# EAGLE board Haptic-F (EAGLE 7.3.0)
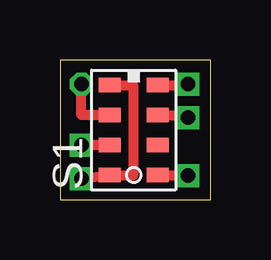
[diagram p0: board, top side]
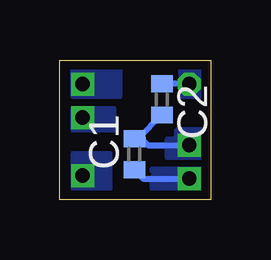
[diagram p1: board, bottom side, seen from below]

Size 6.27 x 5.83 mm. Coordinates in mm from the lower left corner, seen from the top.
Outline: 0,0 6.27,0 6.27,5.83 0,5.83 0,0
Copper layers (1*16): Top 0.0356mm / dielectric 1.5011mm / Bottom 0.0356mm
Design rules "LaenPCBOrder": minimum track width 6mil, minimum drill 13mil, track to track 6mil, track to pad 6mil, pad to pad 6mil, via to via 6mil, smd to smd 6mil, copper to edge 15mil, drill to drill 6mil, minimum pad ring 7mil, minimum via ring 7mil, stop-mask expansion 3mil, vias tented up to drill 0mil, thermal gap 10mil
Net classes: 0 default: width 0.127 mm, drill 0.508 mm, clearance 0.254 mm

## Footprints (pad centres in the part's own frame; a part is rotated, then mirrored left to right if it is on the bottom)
C0402 = smd 0.7 x 0.9: 1 -0.65,0; 2 0.65,0
LGA8 = smd 0.9 x 0.6: 1 -2.5,2.5; 2 -2.5,1.25; 3 -2.5,0; 4 -2.5,-1.25; 5 -0.5,-1.25; 6 -0.5,0; 7 -0.5,1.25; 8 -0.5,2.5

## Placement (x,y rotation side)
C1  1uf  [C0402]  3.17,1.9 90 bottom
C2  1uf  [C0402]  2.03,4.19 270 bottom
S1  MPL115A2  [LGA8]  4.57,2.29 0 top

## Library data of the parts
C1 C2 = eagle-ltspice; SPICEMODEL: NONE; SPICEPREFIX: C
S1 = Youritronics

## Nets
CAP: C2.1 S1.2
GND: C1.2 C2.2 S1.3
RST: S1.5
SCL: S1.8
SDA: S1.7
VDD: C1.1 S1.1 S1.4

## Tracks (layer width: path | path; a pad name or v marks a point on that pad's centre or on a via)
CAP  (via drill 0.6)
  Top 0.406: S1.2 0.89,3.54 v0.89,4.83
  Bottom 0.254: 0.9,4.84 C2.1
  Bottom 0.406: v0.89,4.83 0.9,4.84
  pour Bottom: 0.38,5.33 0.38,4.32 1.4,4.32 1.4,5.33
GND  (via drill 0.6)
  Top 0.406: S1.3 v0.89,2.29
  Bottom 0.254: C2.2 3.02,2.56 C1.2 | 2.89,2.56 2.62,2.29 v0.89,2.29
  Bottom 0.406: 2.89,2.56 C1.2
  pour Bottom: 1.27,2.92 0.38,2.92 0.38,1.78 1.78,1.78 1.78,2.54 1.52,2.54 1.4,2.54 1.4,2.92
RST  (via drill 0.6)
  Top 0.406: S1.5 5.46,1.04 v5.33,1.02
  pour Bottom: 5.71,0.51 4.19,0.51 4.19,1.9 5.71,1.9
SCL  (via drill 0.6)
  Top 0.406: S1.8 5.46,4.79 v5.33,4.83
  pour Bottom: 5.71,4.32 5.71,5.46 3.81,5.46 3.81,4.32
SDA  (via drill 0.6)
  Top 0.406: S1.7 5.46,3.54 v5.33,3.43
  pour Bottom: 5.71,3.81 4.06,3.81 4.06,2.92 5.71,2.92
VDD  (via drill 0.6)
  Top 0.406: S1.1 3.05,4.79 3.05,1.02 2.07,1.02 | 2.07,1.02 S1.4 | 2.07,1.02 v0.89,0.89
  Bottom 0.254: C1.1 2.81,0.89 v0.89,0.89
  pour Bottom: 2.41,1.27 0.38,1.27 0.38,0.51 2.41,0.51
